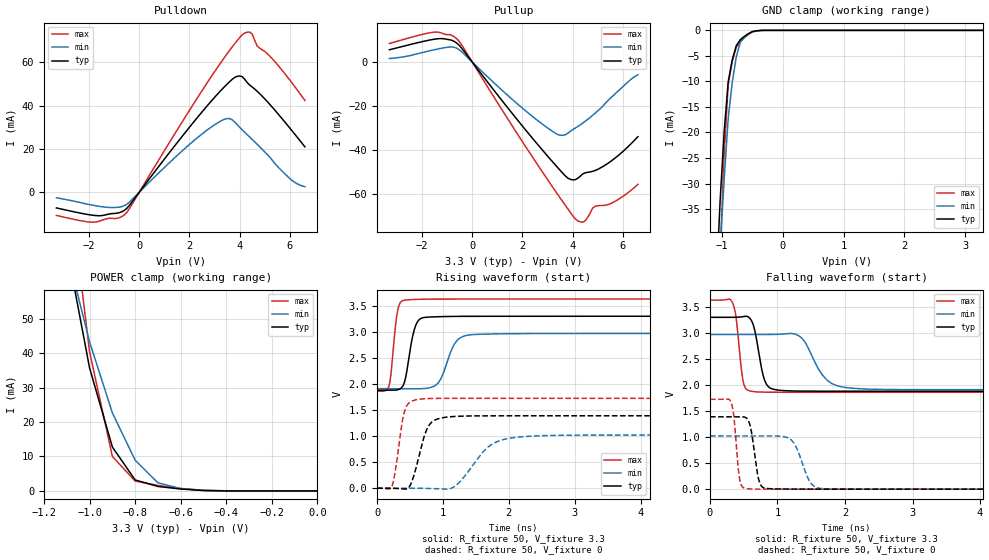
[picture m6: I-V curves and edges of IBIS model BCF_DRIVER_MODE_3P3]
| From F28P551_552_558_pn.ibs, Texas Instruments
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|   Model Cell BCF_DRIVER_MODE_3P3
|BCF_DRIVER_MODE_3P3
[Model]   BCF_DRIVER_MODE_3P3
Model_type   I/O
Polarity   Non-Inverting
Enable   Active-Low
Vinl =  0.8
Vinh =  2
Cref =  15.0000pF
Rref =  100.0000M
Vref =  0V
Vmeas =  1.65
C_comp   1.28683p   1.00698p   1.46241p
[Model Spec]
Vinl   0.8   0.8   0.8
Vinh   2   2   2
[Temperature Range]   25   155   -40
[Voltage Range]   3.3   2.97   3.63
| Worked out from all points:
|   slope of the pulldown table from 0 to 0.495 V, typ, clamps not added: 64.9 ohm
|   slope of the pullup table from 0 to 0.495 V, typ, clamps not added: 67.2 ohm
|   GND clamp passes 1 mA (typ) near -0.61 V on its own axis
|   POWER clamp passes 1 mA (typ) near -0.66 V on its own axis
|   rising waveform, R_fixture 50, V_fixture 3.3: 20-80 % time 120ps typ, 194ps min, 82.1ps max; typ from 1.88 V to 3.3 V
|   rising waveform, R_fixture 50, V_fixture 0: 20-80 % time 182ps typ, 402ps min, 120ps max; typ from 0 V to 1.39 V
|   falling waveform, R_fixture 50, V_fixture 3.3: 20-80 % time 123ps typ, 279ps min, 85.5ps max; typ from 3.3 V to 1.88 V
|   falling waveform, R_fixture 50, V_fixture 0: 20-80 % time 93.4ps typ, 182ps min, 68.6ps max; typ from 1.39 V to 0 V
| Nom Voltages:
|   BIASFET=3.3, VDD=1.2, VDDS=3.3, VSS=0
| Min Voltages:
|   BIASFET=2.97, VDD=1.08, VDDS=2.97, VSS=0
| Max Voltages:
|   BIASFET=3.63, VDD=1.32, VDDS=3.63, VSS=0
[POWER_clamp]
|   voltage   I(typ)   I(min)   I(max)
-3.3V     1.107A     1.023A     1.677A
-1.067V   59.02mA    60.84mA    76.78mA
-1.033V   47.37mA    52.05mA    58.58mA
-1V       35.71mA    43.25mA    40.39mA
-900mV    12.76mA    22.68mA    10.02mA
-800mV    3.185mA    8.924mA    2.863mA
-700mV    1.299mA    2.365mA    1.605mA
-600mV    555.7uA    687.9uA    691.3uA
-500mV    122.7uA    198.2uA    132.8uA
-400mV    9.333uA    32.77uA    7.232uA
0V        319.4pA    4.383nA    281.3pA
[Pulldown]
|   voltage   I(typ)   I(min)   I(max)
-3.3V     -7.269mA   -2.599mA   -10.72mA
-1.8V     -10.73mA   -6.135mA   -13.87mA
-600mV    -8.437mA   -6.22mA    -10.54mA
1.8V      27.16mA    20.04mA    34.19mA
3.1V      45.15mA    31.92mA    57.43mA
3.6V      51.13mA    34.03mA    65.62mA
3.9V      53.6mA     31.29mA    70.12mA
4.2V      52.27mA    27.73mA    73.65mA
4.5V      48.65mA    24.4mA     73.15mA
4.7V      46.65mA    22.12mA    67.59mA
6V        29.63mA    6.308mA    51.82mA
6.6V      20.97mA    2.537mA    42.46mA
[Pullup]
|   voltage   I(typ)   I(min)   I(max)
-3.3V     5.574mA    1.597mA    8.409mA
-1.5V     10.38mA    5.614mA    13.57mA
-900mV    10.12mA    6.83mA     12.44mA
-600mV    8.438mA    6.156mA    10.4mA
1.8V      -26.22mA   -18.96mA   -32.58mA
3.3V      -46.49mA   -32.16mA   -58.26mA
3.8V      -52.53mA   -32.33mA   -66.39mA
4.2V      -52.68mA   -29.22mA   -71.93mA
4.5V      -50.21mA   -26.84mA   -71.95mA
4.9V      -49.12mA   -23.12mA   -65.36mA
5.4V      -45.93mA   -17.52mA   -64.62mA
6.6V      -33.82mA   -5.748mA   -55.41mA
[GND_clamp]
|   voltage   I(typ)   I(min)   I(max)
-3.3V     -944.5mA   -826.8mA   -1.736A
-1.1V     -50.69mA   -57.85mA   -68.88mA
-1.033V   -33.47mA   -42.7mA    -43.81mA
-966.7mV  -19.93mA   -29.17mA   -24.39mA
-900mV    -10.08mA   -17.27mA   -10.63mA
-833.3mV  -5.761mA   -10.17mA   -6.106mA
-766.7mV  -3.004mA   -5.18mA    -3.306mA
-700mV    -1.81mA    -2.304mA   -2.225mA
-566.7mV  -643.8uA   -724.5uA   -783.6uA
-500mV    -225.6uA   -318.6uA   -255.2uA
-300mV    -598.1nA   -5.157uA   -296.9nA
3.3V      319.4pA    6.726uA    227.5pA
[Ramp]
| variable   typ   min   max
dV/dt_f 0.86436924/0.12481639n 0.64790588/0.28264387n  1.0742445/86.811408p
dV/dt_r 0.84453606/0.18452994n 0.62407012/0.40797136n  1.0440117/0.12085082n
R_load = 50
[Rising Waveform]
R_fixture = 50
V_fixture = 3.3
V_fixture_min = 2.97
V_fixture_max = 3.63
|   time   V(typ)   V(min)   V(max)
0s        1.881V     1.91V      1.86V
178.3ps   1.88V      1.91V      1.948V
316.8ps   1.889V     1.91V      3.431V
468.7ps   2.377V     1.909V     3.615V
564.3ps   3.036V     1.908V     3.622V
665.5ps   3.258V     1.909V     3.627V
920ps     3.291V     2.007V     3.63V
1.215ns   3.298V     2.836V     3.63V
1.529ns   3.299V     2.954V     3.63V
20.01ns   3.3V       2.97V      3.63V
[Rising Waveform]
R_fixture = 50
V_fixture = 0
V_fixture_min = 0
V_fixture_max = 0
|   time   V(typ)   V(min)   V(max)
0s        0V         0V         0V
232.7ps   0V         0V         53.33mV
390.8ps   -15.16mV   0V         1.329V
483.7ps   13.77mV    0V         1.633V
711ps     971.7mV    -2.061mV   1.716V
834.9ps   1.273V     -6.405mV   1.722V
1.025ns   1.359V     -17.85mV   1.725V
1.765ns   1.389V     861.4mV    1.725V
2.5ns     1.39V      1.008V     1.725V
20.03ns   1.39V      1.021V     1.725V
[Falling Waveform]
R_fixture = 50
V_fixture = 3.3
V_fixture_min = 2.97
V_fixture_max = 3.63
|   time   V(typ)   V(min)   V(max)
0s        3.3V       2.97V      3.63V
322.4ps   3.3V       2.97V      3.61V
377ps     3.301V     2.97V      3.38V
501.4ps   3.316V     2.97V      2.018V
673.1ps   2.988V     2.97V      1.871V
834.1ps   2.019V     2.97V      1.863V
1.142ns   1.889V     2.987V     1.861V
1.735ns   1.882V     2.092V     1.861V
2.229ns   1.881V     1.928V     1.861V
20.01ns   1.881V     1.91V      1.861V
[Falling Waveform]
R_fixture = 50
V_fixture = 0
V_fixture_min = 0
V_fixture_max = 0
|   time   V(typ)   V(min)   V(max)
0s        1.39V      1.021V     1.725V
305.2ps   1.39V      1.021V     1.692V
442.5ps   1.392V     1.021V     171.1mV
575.8ps   1.293V     1.021V     6.223mV
719.9ps   190.6mV    1.022V     0V
878.5ps   9.487mV    1.023V     0V
1.203ns   0V         948.6mV    0V
1.474ns   0V         153.1mV    0V
1.692ns   0V         9.187mV    0V
20.03ns   0V         0V         0V
